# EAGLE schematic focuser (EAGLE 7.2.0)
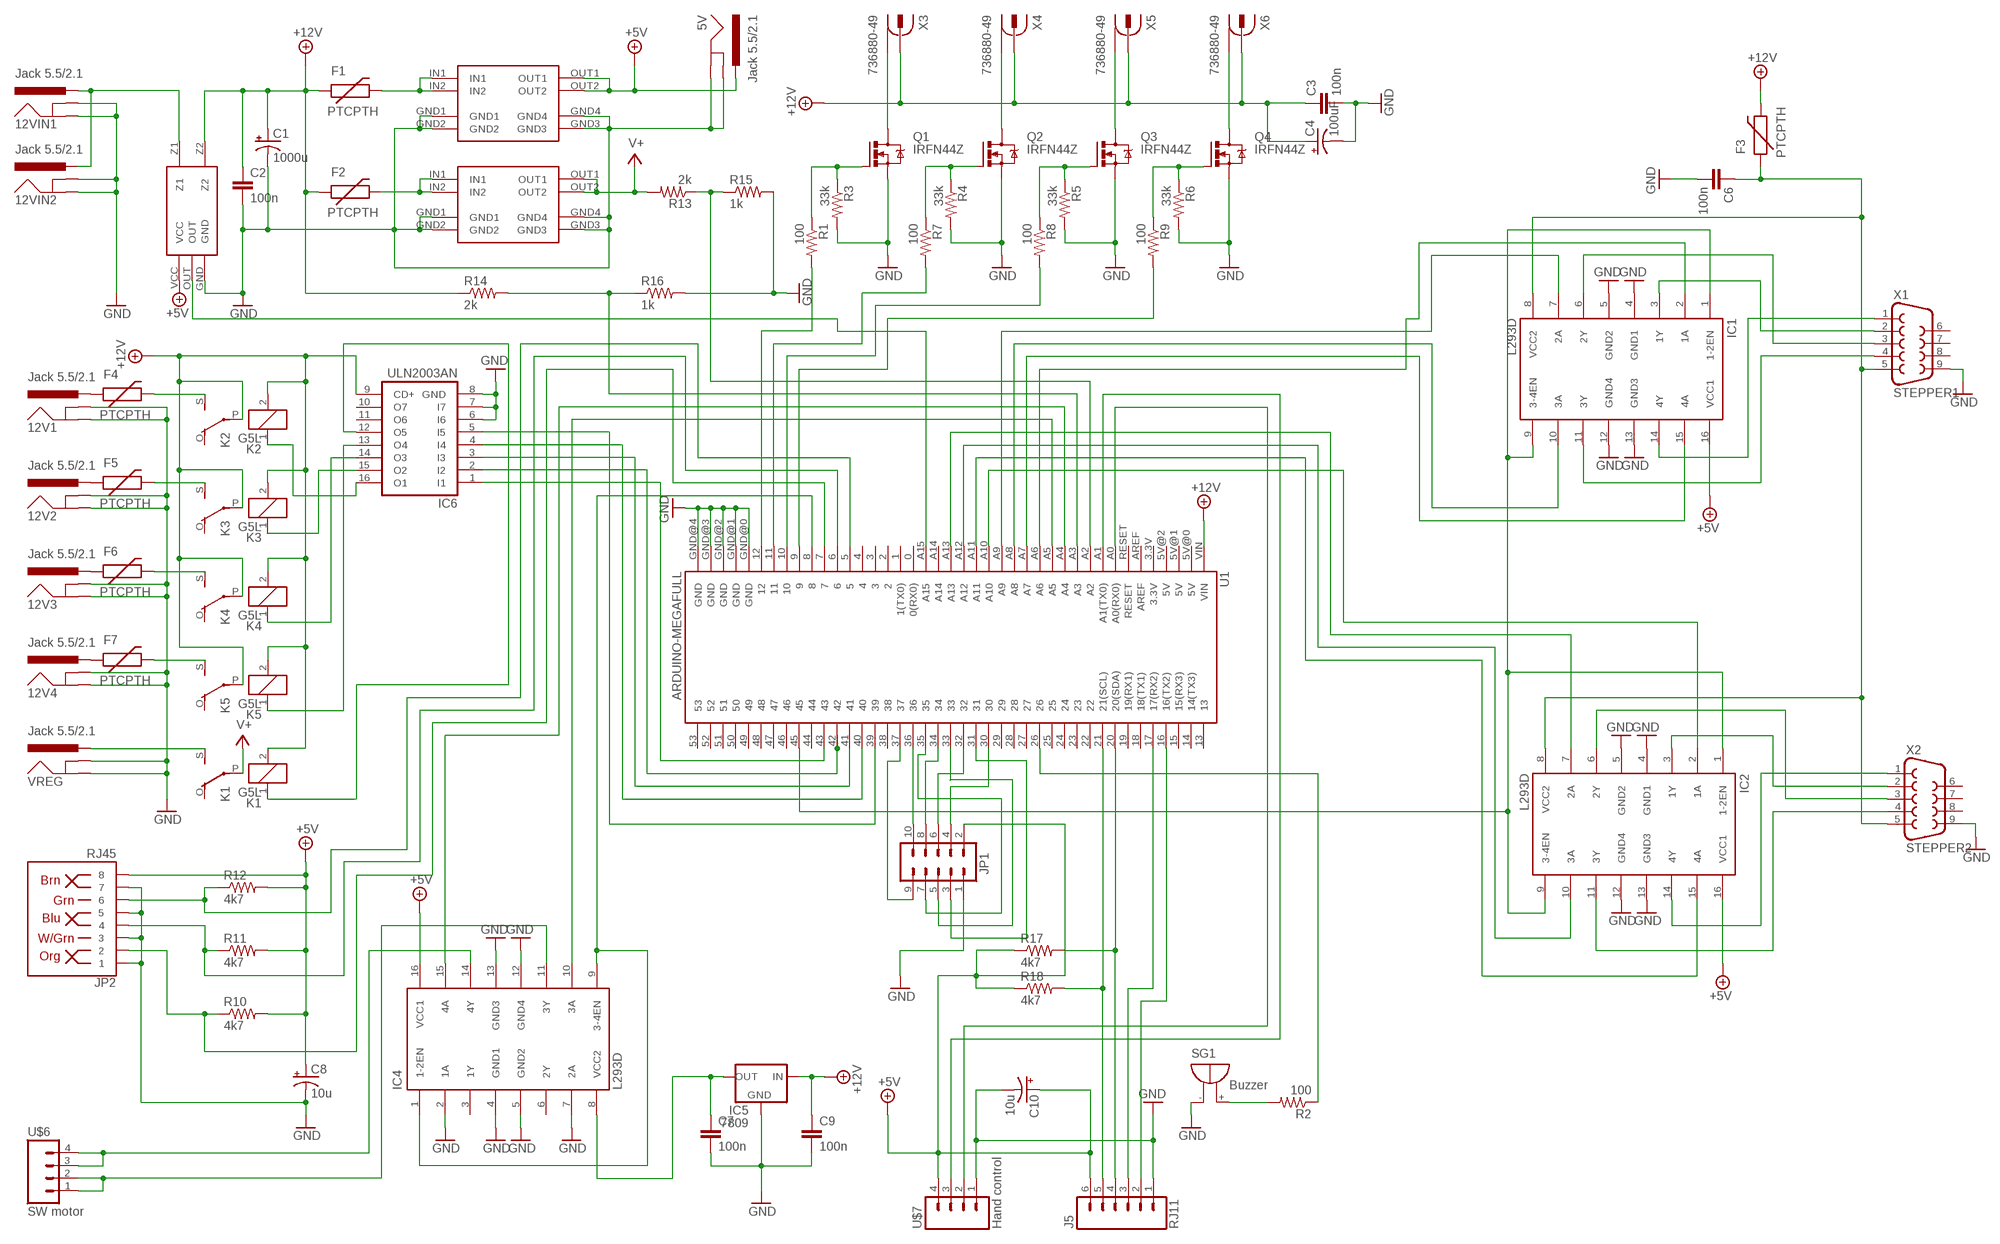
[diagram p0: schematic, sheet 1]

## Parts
5V  Jack 5.5/2.1  POWER_JACKPTH  [POWER_JACK_PTH]
12V1  Jack 5.5/2.1  POWER_JACKPTH  [POWER_JACK_PTH]
12V2  Jack 5.5/2.1  POWER_JACKPTH  [POWER_JACK_PTH]
12V3  Jack 5.5/2.1  POWER_JACKPTH  [POWER_JACK_PTH]
12V4  Jack 5.5/2.1  POWER_JACKPTH  [POWER_JACK_PTH]
12VIN1  Jack 5.5/2.1  POWER_JACKPTH  [POWER_JACK_PTH]
12VIN2  Jack 5.5/2.1  POWER_JACKPTH  [POWER_JACK_PTH]
C1  1000u  CAP_POLPTH4  [CPOL-RADIAL-1000UF-25V]
C2  100n  CAPPTH1  [CAP-PTH-5MM]
C3  100n  CAPPTH1  [CAP-PTH-5MM]
C4  100uF  CAP_POLPTH1  [CPOL-RADIAL-100UF-25V]
C6  100n  CAPPTH1  [CAP-PTH-5MM]
C7  100n  CAPPTH1  [CAP-PTH-5MM]
C8  10u  CAP_POLPTH2  [CPOL-RADIAL-10UF-25V]
C9  100n  CAPPTH1  [CAP-PTH-5MM]
C10  10u  CAP_POLPTH2  [CPOL-RADIAL-10UF-25V]
F1  PTCPTH  [PTC]
F2  PTCPTH  [PTC]
F3  PTCPTH  [PTC]
F4  PTCPTH  [PTC]
F5  PTCPTH  [PTC]
F6  PTCPTH  [PTC]
F7  PTCPTH  [PTC]
IC1  L293D  [DIL16]
IC2  L293D  [DIL16]
IC4  L293D  [DIL16]
IC5  7809  V_REG_78XXSINK  [TO220-IGO]
IC6  ULN2003AN  [DIL16]
J5  RJ11  RJ11-6PTH  [RJ11-6]
JP1  M05X2PTH  [AVR_ICSP]
JP2  RJ45  RJ45-8PTH  [RJ45-8]
K1  G5L  [G5LE]
K2  G5L  [G5LE]
K3  G5L  [G5LE]
K4  G5L  [G5LE]
K5  G5L  [G5LE]
Q1  IRFN44Z  IRF540  [TO220BV]
Q2  IRFN44Z  IRF540  [TO220BV]
Q3  IRFN44Z  IRF540  [TO220BV]
Q4  IRFN44Z  IRF540  [TO220BV]
R1  100  RESISTORPTH1  [AXIAL-0.3]
R2  100  RESISTORPTH1  [AXIAL-0.3]
R3  33k  RESISTORPTH1  [AXIAL-0.3]
R4  33k  RESISTORPTH1  [AXIAL-0.3]
R5  33k  RESISTORPTH1  [AXIAL-0.3]
R6  33k  RESISTORPTH1  [AXIAL-0.3]
R7  100  RESISTORPTH1  [AXIAL-0.3]
R8  100  RESISTORPTH1  [AXIAL-0.3]
R9  100  RESISTORPTH1  [AXIAL-0.3]
R10  4k7  RESISTORPTH1  [AXIAL-0.3]
R11  4k7  RESISTORPTH1  [AXIAL-0.3]
R12  4k7  RESISTORPTH1  [AXIAL-0.3]
R13  2k  RESISTORPTH1  [AXIAL-0.3]
R14  2k  RESISTORPTH1  [AXIAL-0.3]
R15  1k  RESISTORPTH1  [AXIAL-0.3]
R16  1k  RESISTORPTH1  [AXIAL-0.3]
R17  4k7  RESISTORPTH1  [AXIAL-0.3]
R18  4k7  RESISTORPTH1  [AXIAL-0.3]
SG1  Buzzer  F/QMBIII  [F/QMBIII]
U1  ARDUINO-MEGAFULL  [ARDUINO_MEGA]
U$1  MP1584-BUCK  [DCDC-1584]
U$2  MP1584-BUCK  [DCDC-1584]
U$3  ASC712  [ASC712]
U$6  SW motor  RJ9PTH  [RJ9]
U$7  Hand control  RJ9PTH  [RJ9]
VREG  Jack 5.5/2.1  POWER_JACKPTH  [POWER_JACK_PTH]
X1  STEPPER1  DB9  [DB9]
X2  STEPPER2  DB9  [DB9]
X3  736880-49  [736880-49]
X4  736880-49  [736880-49]
X5  736880-49  [736880-49]
X6  736880-49  [736880-49]

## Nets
+5V: 5V.PWR C8.1(+) C10.1(+) IC1.16(VCC1) IC2.16(VCC1) IC4.16(VCC1) J5.6 JP1.2 JP2.8 R10.P$2 R11.P$2 R12.P$2 R17.P$1 R18.P$1 U$1.OUT1 U$1.OUT2 U$3.VCC U$7.4
+12V: C1.1(+) C2.1 C3.1 C4.1(+) C9.1 F1.P$1 F2.P$1 F3.P$2 IC5.IN IC6.9(CD+) K1.2 K2.2 K2.P(2:P) K3.2 K3.P(2:P) K4.2 K4.P(2:P) K5.2 K5.P(2:P) R14.P$1 U1.VIN U$3.Z2 X3.2 X4.2 X5.2 X6.2
GND: 5V.GND 5V.GNDBREAK 12V1.GND 12V1.GNDBREAK 12V2.GND 12V2.GNDBREAK 12V3.GND 12V3.GNDBREAK 12V4.GND 12V4.GNDBREAK 12VIN1.GND 12VIN1.GNDBREAK 12VIN2.GND 12VIN2.GNDBREAK C1.2(-) C2.2 C3.2 C4.2(-) C6.2 C7.2 C8.2(-) C9.2 C10.2(-) IC1.4(GND1) IC1.5(GND2) IC1.12(GND4) IC1.13(GND3) IC2.4(GND1) IC2.5(GND2) IC2.12(GND4) IC2.13(GND3) IC4.2(1A) IC4.4(GND1) IC4.5(GND2) IC4.7(2A) IC4.12(GND4) IC4.13(GND3) IC5.GND IC6.6(I6) IC6.7(I7) IC6.8(GND) J5.1 JP1.1 JP2.1 JP2.3 JP2.5 JP2.7 Q1.S Q2.S Q3.S Q4.S R3.P$2 R4.P$2 R5.P$2 R6.P$2 R15.P$2 R16.P$2 SG1.-(+) U1.GND@0(GND) U1.GND@1(GND) U1.GND@2(GND) U1.GND@3(GND) U1.GND@4(GND) U$1.GND1 U$1.GND2 U$1.GND3 U$1.GND4 U$2.GND1 U$2.GND2 U$2.GND3 U$2.GND4 U$3.GND U$7.1 VREG.GND VREG.GNDBREAK X1.9 X2.9
N$1: J5.4 R17.P$2 U1.20(20(SDA))
N$2: J5.5 R18.P$2 U1.21(21(SCL))
N$3: C7.1 IC4.8(VCC2) IC5.OUT
N$4: IC2.14(4Y) X2.1
N$5: IC1.3(1Y) X1.2
N$6: IC1.14(4Y) X1.1
N$7: IC1.11(3Y) X1.4
N$8: F4.P$2 K2.S(2:S)
N$9: F5.P$2 K3.S(2:S)
N$10: R9.P$2 U1.9
N$11: R8.P$2 U1.10
N$12: IC1.1(1-2EN) IC1.9(3-4EN) IC2.1(1-2EN) IC2.9(3-4EN) U1.45
N$13: J5.3 U1.17(17(RX2))
N$14: R7.P$2 U1.11
N$15: IC2.6(2Y) X2.3
N$16: IC1.6(2Y) X1.3
N$17: J5.2 U1.16(16(TX2))
N$18: IC6.4(I4) U1.40
N$19: F6.P$2 K4.S(2:S)
N$20: F7.P$2 K5.S(2:S)
N$21: IC6.5(I5) U1.39
N$22: R13.P$1 R15.P$1 U1.A2
N$23: IC4.15(4A) U1.A4
N$24: R2.P$2 SG1.+(-)
N$25: IC6.2(I2) U1.42
N$26: 12VIN1.PWR 12VIN2.PWR U$3.Z1
N$27: IC6.1(I1) U1.43
N$28: F2.P$2 U$2.IN1 U$2.IN2
N$29: IC6.3(I3) U1.41
N$30: IC4.1(1-2EN) IC4.9(3-4EN) U1.8
N$31: IC4.10(3A) U1.A5
N$32: U1.A15 U$3.OUT
N$33: IC1.7(2A) U1.A9
N$34: U1.A0(A0(RX0)) U$7.2
N$35: Q1.D X3.1 X3.1@1 X3.1@2
N$36: Q2.D X4.1 X4.1@1 X4.1@2
N$37: K1.S(2:S) VREG.PWR
N$38: Q3.D X5.1 X5.1@1 X5.1@2
N$39: Q4.G R6.P$1 R9.P$1
N$40: Q3.G R5.P$1 R8.P$1
N$41: Q2.G R4.P$1 R7.P$1
N$42: Q1.G R1.P$1 R3.P$1
N$43: 12V1.PWR F4.P$1
N$44: U1.A1(A1(TX0)) U$7.3
N$45: IC4.14(4Y) U$6.3 U$6.4
N$46: R2.P$1 U1.26
N$47: R14.P$2 R16.P$1 U1.A3
N$48: IC1.10(3A) U1.A8
N$49: IC1.15(4A) U1.A7
N$50: IC1.2(1A) U1.A6
N$51: IC4.11(3Y) U$6.1 U$6.2
N$52: 12V2.PWR F5.P$1
N$53: JP1.10 U1.36
N$54: IC6.14(O3) K4.1
N$55: IC6.13(O4) K5.1
N$56: IC6.15(O2) K3.1
N$57: IC6.16(O1) K2.1
N$58 [power]: C6.1 F3.P$1 IC1.8(VCC2) IC2.8(VCC2) X1.5 X2.5
N$59: JP2.6 R12.P$1 U1.5
N$60: 12V3.PWR F6.P$1
N$61: 12V4.PWR F7.P$1
N$62: JP1.8 U1.34
N$63: IC6.12(O5) K1.1
N$64: Q4.D X6.1 X6.1@1 X6.1@2
N$65: JP2.4 R11.P$1 U1.6
N$66: JP1.6 U1.32
N$67: JP1.4 U1.30
N$68: JP1.9 U1.37
N$69: F1.P$2 U$1.IN1 U$1.IN2
N$70: JP1.7 U1.35
N$71: JP2.2 R10.P$1 U1.7
N$72: JP1.5 U1.33
N$73: IC2.11(3Y) X2.4
N$74: JP1.3 U1.31
N$79: R1.P$2 U1.12
N$80: IC2.3(1Y) X2.2
N$81: IC2.7(2A) U1.A13
N$82: IC2.10(3A) U1.A12
N$83: IC2.15(4A) U1.A11
N$84: IC2.2(1A) U1.A10
V+: K1.P(2:P) R13.P$2 U$2.OUT1 U$2.OUT2
Unconnected: IC4.3(1Y) IC4.6(2Y) IC6.10(O7) IC6.11(O6) K1.O(2:O) K2.O(2:O) K3.O(2:O) K4.O(2:O) K5.O(2:O) U1.0(0(RX0)) U1.1(1(TX0)) U1.2 U1.3 U1.3.3V U1.4 U1.5V@0(5V) U1.5V@1(5V) U1.5V@2(5V) U1.13 U1.14(14(TX3)) U1.15(15(RX3)) U1.18(18(TX1)) U1.19(19(RX1)) U1.22 U1.23 U1.24 U1.25 U1.27 U1.28 U1.29 U1.38 U1.44 U1.46 U1.47 U1.48 U1.49 U1.50 U1.51 U1.52 U1.53 U1.A14 U1.AREF U1.RESET X1.6 X1.7 X1.8 X2.6 X2.7 X2.8

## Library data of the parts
5V 12V1-12V4 12VIN1 12VIN2 VREG = SparkFun-Connectors:POWER_JACK: Power Jack This is the standard 5.5mm barrel jack for power. The PTH is the most common, proven, reliable, footprint. The Slot footprint only works if the mill layer is transmitted to the PCB fab house so be warned. Mating wall wart : TOL-00298 (and others); PROD_ID: CONN-08197
C1 C8 C10 = SparkFun:CAP_POL: Capacitor Polarized
C2 C3 C6 C7 C9 = SparkFun:CAP: Capacitor
C4 = SparkFun-Passives:CAP_POL: Capacitor Polarized
F1-F7 = SparkFun:PTC: Resettable Fuse PTC
IC1 IC2 IC4 = st-microelectronics:L293D: PUSH-PULL 4 CHANNEL DRIVER; MPN: L293D; OC_FARNELL: 9589619; OC_NEWARK: 56P8249
IC5 = SparkFun-PowerIC:V_REG_78XX: Voltage Regulator Standard 78xx regulator. IGO (Input Ground Output). Spark Fun Electronics SKU : COM-00107
IC6 = uln-udn:ULN2003A: DRIVER ARRAY
J5 = SparkFun-Connectors:RJ11-6: RJ11 Jack Simple 6 pin RJ11 jack. Commonly found on CAT3 devices and Microchip programmers. SKU: PRT-00132; PROD_ID: CONN-08590
JP1 = SparkFun-Connectors:M05X2: Header 5x2 Standard 10-pin dual row 0.1" header. Commonly used with AVR-ISP. Use with Spark Fun Electronics SKU: PRT-00778
JP2 = SparkFun-Connectors:RJ45-8: RJ45 Jack Simple RJ45, 8-pin connection - connector for common Cat5, Cat5e, and Cat6 Ethernet cables. Footprint not yet proven in production. Connector sku is PRT-00643; Breakout PCB sku is BOB-00716.; PROD_ID: CONN-08506
K1-K5 = relay:G5L: RELAY 1 x switch, 10 A/120 V AC, 8 A/30 V ADC, Omron; OC_FARNELL: unknown; OC_NEWARK: unknown
Q1-Q4 = transistor-power:IRF540: HEXFET Power MOSFET
R1-R18 = SparkFun:RESISTOR: Resistor
SG1 = buzzer2:F/QMBIII: BUZZER; OC_FARNELL: unknown; OC_NEWARK: unknown
U1 = SparkFun-Boards:ARDUINO-MEGA: Arduino Mega board footprint
U$1 U$2 = jolo-lib:MP1584-BUCK
U$3 = jolo-lib:ASC712
U$6 U$7 = SparkFun:RJ9
X1 X2 = SparkFun:DB9: DB9 Connector Standard DB9 (D-Sub 9) serial connector. Can be used for CAN bus as well as RS485 and RS232. Footprint production proven. Spark Fun Electronics SKU : PRT-00429
X3-X6 = con-conrad:736880-49: Cinch Connector ( RCA Jack )

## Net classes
0 default: width 0.254 mm, drill 0.635 mm, clearance 0.203 mm
1 power: width 0.254 mm, drill 0.635 mm, clearance 0.203 mm

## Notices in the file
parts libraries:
SparkFun: Licensing: CC v3.0 Share-Alike You are welcome to use this library for commercial purposes.
SparkFun-Boards: Licensing: Creative Commons ShareAlike 4.0 International - https://creativecommons.org/licenses/by-sa/4.0
